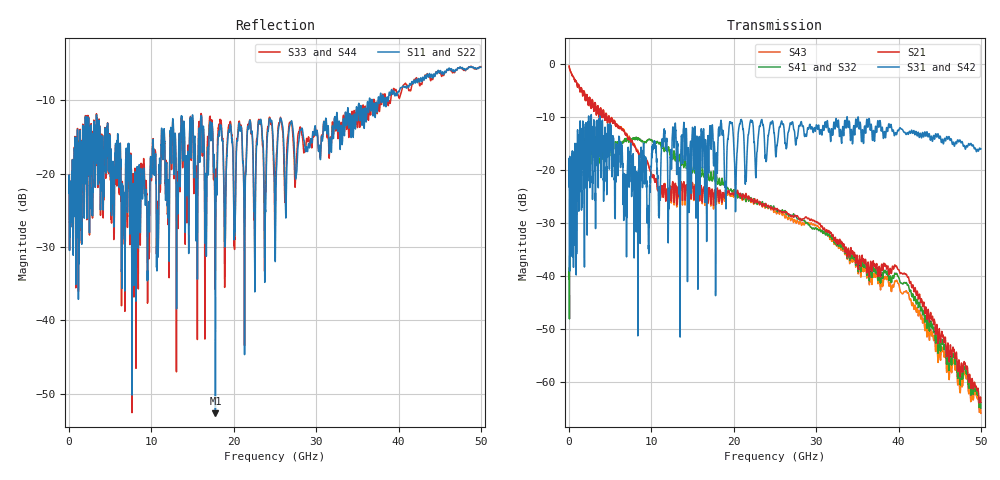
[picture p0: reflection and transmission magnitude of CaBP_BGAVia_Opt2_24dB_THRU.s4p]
!* Samtec Inc. NovaRay Examax Flyover System  *
!*  REV DATE  = 08/08/18  *
!*  TYPE  = TOUCHSTONE  *
!*  PORTS  = 4 port  *
!*  UNITS  = GHz  *
!*  DATA RANGE = DC  to 50 GHz; 10 MHz Step  *
!*  PARAMETER  = S  *
!*  FORMAT  = Real-Imaginary  *
!*  REFERENCE  = 50 ohms  *
!*  SOURCE  = HFSS  *
!*  VALIDATED  = No  *
!*  MANUFACTURER = SAMTEC  *
!*  INTERCONNECT = NVAx to EBCx to EBCx to NVAx  *
!*  [Full Channel NVAx to EBCx to EBCx to NVAx  with PCB Trace and BGA Via]  *
!*  BOUNDARY A  = Silicon BGA Ball Pad  *
!*  BOUNDARY B  = Silicon BGA Ball Pad  *
!*  NVAx (end a) ->>- (end b) NVAx  *
!*  Port 01 ->>- Port 02  *
!*  Port 03 ->>- Port 04  *
!***************************** CHANNEL MODEL ******************************************
# GHz S RI R 50
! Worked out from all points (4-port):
!   5000 points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, 10 MHz to 50 GHz, reference 50 ohm
!   strongest paths, dB at 10 MHz, 12.51 GHz, 25.01 GHz, 37.51 GHz, 50 GHz:
!     S31: -23.2, -14.5, -15.2, -10.7, -16.0
!     S42: -23.2, -14.5, -15.2, -10.7, -16.0
!     S21: -0.4, -23.1, -27.3, -40.1, -63.9
!     S41: -40.6, -17.3, -27.4, -40.8, -64.9
!     S32: -40.6, -17.3, -27.4, -40.8, -64.9
!     S43: -0.4, -23.5, -27.8, -41.5, -65.9
!   lowest |S11| = -52.7 dB at 17.77 GHz (marker M1), VSWR 1.00, Z = 49.8 - j0.145 ohm
!   |S11| at or under -10 dB: start of sweep to 36.46 GHz; 36.55 GHz to 36.75 GHz (204 MHz wide, 0.557 % of centre); 36.79 GHz to 37.51 GHz (722.9 MHz wide, 1.95 % of centre)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
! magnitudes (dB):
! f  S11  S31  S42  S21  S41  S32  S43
! 10 MHz  -22.7  -23.2  -23.2  -0.4  -40.6  -40.6  -0.4
! 780 MHz  -17.3  -18.6  -18.6  -3.2  -20.4  -20.4  -3.2
! 2.12 GHz  -15.3  -15.8  -15.8  -6.0  -16.8  -16.8  -6.0
! 17.22 GHz  -15.5  -15.4  -15.4  -26.4  -20.3  -20.3  -26.7
! 17.77 GHz  -52.7  -28.1  -28.1  -24.2  -21.8  -21.8  -25.0
! 39.75 GHz  -9.2  -13.3  -13.3  -38.1  -39.5  -39.5  -40.8
! 50 GHz  -5.5  -16.0  -16.0  -63.9  -64.9  -64.9  -65.9
